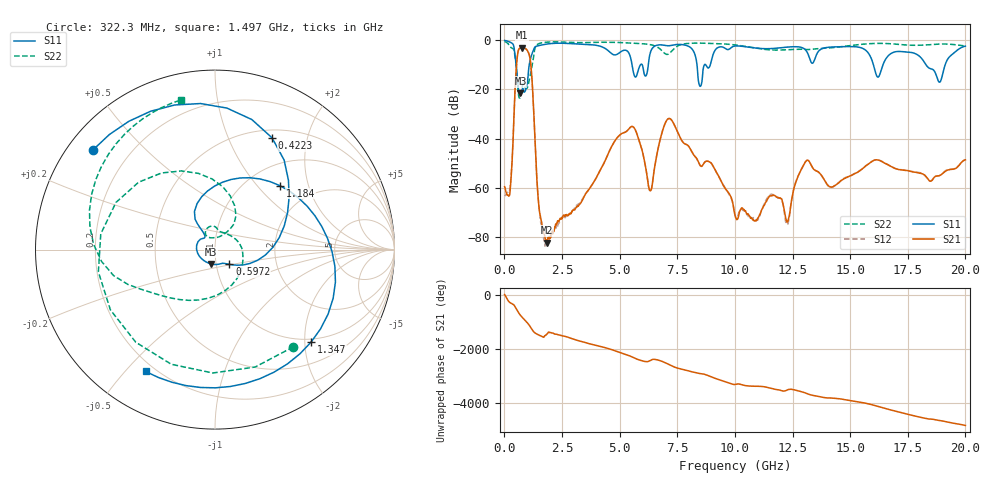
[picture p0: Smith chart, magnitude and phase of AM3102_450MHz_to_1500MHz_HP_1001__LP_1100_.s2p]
!Agilent Technologies,E8364B,MY43040894,A.07.50.67
!Agilent E8364B: A.07.50.67
!Date: Thursday, January 11, 2018 06:04:37
!Correction: S11(Full 2 Port(1,2))
!S21(Full 2 Port(1,2))
!S12(Full 2 Port(1,2))
!S22(Full 2 Port(1,2))
!S2P File: Measurements: S11, S21, S12, S22:
# Hz S  dB  R 50
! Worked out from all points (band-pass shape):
!   1601 points, 10 MHz to 20 GHz, reference 50 ohm
!   highest |S21| = -2.96 dB at 759.6 MHz (marker M1); lowest = -82.3 dB at 1.834 GHz (marker M2)
!   |S21| within 3 dB of the highest: 570 MHz to 1.08 GHz (510.2 MHz wide, 61.8 % of centre)
!   lowest |S11| = -21.6 dB at 697.2 MHz (marker M3), VSWR 1.18, Z = 47.3 - j7.63 ohm
!   |S11| at or under -10 dB: 511.7 MHz to 1.078 GHz (566.5 MHz wide, 71.3 % of centre); 16.01 GHz to 16.42 GHz (412 MHz wide, 2.54 % of centre); 18.29 GHz to 19.12 GHz (825.5 MHz wide, 4.41 % of centre)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
!   |S22| runs from -23.5 to -0.5 dB; largest |S21 - S12| = 0.00063
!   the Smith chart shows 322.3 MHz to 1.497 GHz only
!   S11 on the Smith chart (normalised r, x): 322.3 MHz: 0.07, +0.35; 422.3 MHz: 0.60, +1.46; 597.2 MHz: 1.16, -0.19; 1.184 GHz: 1.39, +1.33; 1.347 GHz: 0.93, -2.14; 1.497 GHz: 0.16, -0.57
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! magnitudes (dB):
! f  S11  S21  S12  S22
! 10 MHz  -0.1  -59.6  -63.4  -0.5
! 322.3 MHz  -1.1  -51.3  -50.6  -3.2
! 422.3 MHz  -3.1  -29.3  -29.4  -4.3
! 597.2 MHz  -18.8  -4.4  -4.4  -21.0
! 697.2 MHz  -21.6  -3.1  -3.1  -23.4
! 759.6 MHz  -20.5  -3.0  -3.0  -20.2
! 1.184 GHz  -5.9  -14.1  -14.1  -11.3
! 1.347 GHz  -2.6  -44.7  -44.8  -2.7
! 1.497 GHz  -2.1  -67.5  -67.5  -1.4
! 1.834 GHz  -1.5  -82.3  -82.6  -0.8
! 3.346 GHz  -1.6  -65.7  -65.4  -0.9
! 5.457 GHz  -6.5  -35.4  -35.5  -1.1
! 6.319 GHz  -5.4  -61.2  -61.4  -1.7
! 6.682 GHz  -1.9  -43.4  -43.5  -3.0
! 7.219 GHz  -2.1  -32.1  -32.1  -4.8
! 8.493 GHz  -18.7  -50.9  -50.9  -1.1
! 10.01 GHz  -2.3  -71.3  -71.3  -1.9
! 12.28 GHz  -2.8  -74.0  -74.9  -3.8
! 13.34 GHz  -9.3  -51.4  -51.4  -3.6
! 16.68 GHz  -6.1  -50.9  -50.8  -1.3
! 18.88 GHz  -17.1  -55.1  -55.1  -1.5
! 20 GHz  -2.4  -48.6  -48.5  -2.3
